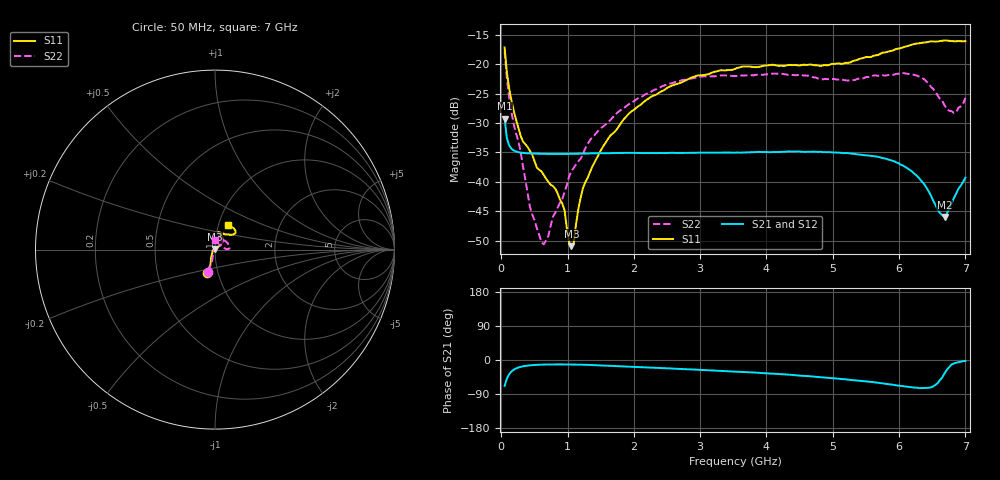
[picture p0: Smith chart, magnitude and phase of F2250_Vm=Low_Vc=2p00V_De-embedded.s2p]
! Integrated Device Technology
! Corporate Headquarters
! 6024 Silver Creek Valley Road
! San Jose, CA 95138  USA
! Phone:  1-408-284-8200
! Toll Free:  1-800-223-1366
! Webpage:  http://www.idt.com/
! Timing and RF Division
! 515 Groton Road, Suite 102
! Westford, MA 01886-6024
! Device:  F2250
! Description: Voltage Variable RF Attenuator
! Frequency:  50.0 -  6000.00 MHz
! Package:  3x3 mm Thin QFN Plastic Package: 16 pin
! Ports:  2 RF, 3 DC
!  Pin  1  = GND
!  Pin  2  = NC
!  Pin  3  = RF1  = Port 1
!  Pin  4  = NC
!  Pin  5  = GND
!  Pin  6  = GND
!  Pin  7  = GND
!  Pin  8  = GND
!  Pin  9  = NC
!  Pin 10  = RF2  = Port 2
!  Pin 11  = NC
!  Pin 12  = GND
!  Pin 13  = GND
!  Pin 14  = VCNTRL
!  Pin 15  = VDD
!  Pin 16  = VMODE
! Vcntrl:  2.000 Volts
! Vmode:  +0.000 Volts
! Vdd:  +3.30  Volts
! Current:  1.181 mA
! Data:  The device was measured on a the F2250 evaluation board which has
!  individual transmission lines to the RF pins.  Data was collected
!  using a calibrated network analyzer.  The evaluation board was
!  de-embedded using a TRL calibration technique.
!  The reference plane is the edge of the package pin.
! Misc:  SN 10
!  Action Tracker AT0258
! Date Measured:  2014-11-26
! Date:  2015-10-15  MJV
! Note:
!  Integrated Device Technology supplies this data as a sample of measured
!  data at the package pin for this product.  Your particular data for this
!  product may vary.
!  Data was taken at 25 degrees C.
!  Integrated Device Technology reserves the right to change this data at anytime.
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# GHz S dB R 50
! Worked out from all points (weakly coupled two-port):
!   201 points, 50 MHz to 7 GHz, reference 50 ohm
!   highest |S21| = -29.27 dB at 50 MHz (marker M1); lowest = -46.0 dB at 6.687 GHz (marker M2)
!   lowest |S11| = -50.9 dB at 1.058 GHz (marker M3), VSWR 1.01, Z = 49.8 + j0.241 ohm
!   |S11| at or under -10 dB: start of sweep to end of sweep
!   |S22| runs from -50.6 to -17.8 dB; largest |S21 - S12| = 6.4e-05
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0.05  -17.18 -108.6  -29.27 -68.2  -29.26 -68.2  -17.82 -108.3
0.1195  -24.20 -111.7  -33.84 -37.3  -33.84 -37.3  -25.82 -106.1
0.29325  -32.21 -127.6  -35.03 -18.0  -35.03 -18.0  -35.01 -111.4
0.43225  -34.74 -144.5  -35.18 -14.0  -35.17 -14.0  -44.25 -137.2
0.606  -38.22 -160.7  -35.24 -12.2  -35.25 -12.2  -50.24 155.5
0.71025  -40.01 -168.3  -35.26 -11.8  -35.26 -11.8  -49.18 103.9
0.77975  -40.72 177.6  -35.27 -11.7  -35.27 -11.7  -45.89 91.0
0.91875  -43.66 158.3  -35.27 -11.7  -35.27 -11.7  -42.94 71.5
1.023  -50.27 143.5  -35.26 -11.8  -35.27 -11.8  -39.09 64.1
1.05775  -50.92 121.8  -35.26 -11.9  -35.26 -11.9  -38.16 61.8
1.0925  -50.50 89.5  -35.25 -12.0  -35.25 -12.0  -37.62 58.1
1.162  -44.62 56.2  -35.23 -12.2  -35.23 -12.2  -36.48 50.3
1.2315  -41.09 43.9  -35.20 -12.5  -35.21 -12.5  -35.29 45.1
1.6485  -32.11 41.9  -35.13 -15.2  -35.13 -15.1  -29.46 44.4
2.37825  -24.87 47.3  -35.10 -21.0  -35.10 -21.0  -24.08 46.3
3.525  -20.81 72.5  -35.04 -30.5  -35.04 -30.5  -22.04 69.2
4.7065  -20.17 72.3  -34.87 -43.7  -34.87 -43.7  -22.25 69.0
5.85325  -17.82 40.4  -36.27 -64.2  -36.26 -64.2  -21.83 17.2
6.33975  -16.40 41.0  -39.90 -74.1  -39.91 -74.1  -22.30 3.1
6.68725  -15.99 48.8  -45.96 -34.5  -45.92 -34.2  -27.02 23.5
6.861  -16.13 55.1  -41.98 -7.1  -41.93 -7.0  -28.15 58.6
7  -16.12 63.2  -39.26 -2.7  -39.22 -2.9  -25.76 87.4
